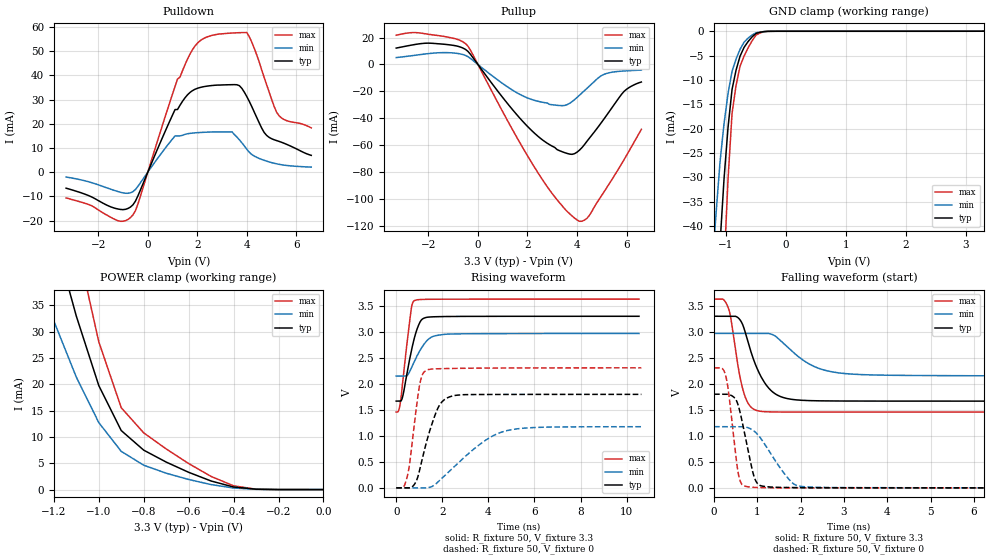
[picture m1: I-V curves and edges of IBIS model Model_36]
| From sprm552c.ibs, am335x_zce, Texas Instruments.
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| Model based on original model for BC1833DV50BPBFBP18LL_SSDHV
|   Sub model BC50B_V_PUPDOFF_10P_3P3
[model]   Model_36
|[Description]  [3.3V-I/O-PI-NORMAL, IND, 10%]
|   NORMAL,Weak pull up/down disabled,Industrial temperature range
|   (-40C to 125C, 25C nominal),10% power supply tolerance
|[Input Load]   PI
|[Output Drive] NORMAL
|Voltage   3.3V
|Mode   I/O
Model_type   I/O
Polarity   Non-Inverting
Enable   Active-Low
Vinl =  0.8V
Vinh =  2V
Cref =  15pF
Rref =  100.0000M
Vref =  0V
Vmeas =  1.65
C_comp   1.841028p   1.702526p   1.921952p
[Model Spec]
Vinl   0.8V   0.8V   0.8V
Vinh   2V   2V   2V
[Temperature Range]   25   125   -40
[Voltage Range]   3.3   2.97   3.63
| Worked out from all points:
|   slope of the pulldown table from 0 to 0.495 V, typ, clamps not added: 41.2 ohm
|   slope of the pullup table from 0 to 0.495 V, typ, clamps not added: 40 ohm
|   GND clamp passes 1 mA (typ) near -0.55 V on its own axis
|   POWER clamp passes 1 mA (typ) near -0.44 V on its own axis
|   rising waveform, R_fixture 50, V_fixture 3.3: 20-80 % time 461ps typ, 616ps min, 332ps max; typ from 1.67 V to 3.3 V
|   rising waveform, R_fixture 50, V_fixture 0: 20-80 % time 692ps typ, 1.86ns min, 386ps max; typ from 0 V to 1.8 V
|   falling waveform, R_fixture 50, V_fixture 3.3: 20-80 % time 464ps typ, 800ps min, 265ps max; typ from 3.3 V to 1.67 V
|   falling waveform, R_fixture 50, V_fixture 0: 20-80 % time 273ps typ, 571ps min, 191ps max; typ from 1.8 V to 0 V
[POWER_clamp]
-3.3V     437.1mA    413.2mA    590.8mA
-1.267V   59.46mA    39.86mA    84.25mA
-1.233V   53.93mA    35.93mA    76.6mA
-1.133V   38.09mA    24.91mA    54.45mA
-1.067V   28.54mA    18.48mA    40.82mA
-1.033V   24.14mA    15.6mA     34.44mA
-1V       19.75mA    12.72mA    28.06mA
-900mV    11.21mA    7.259mA    15.54mA
-800mV    7.487mA    4.633mA    10.77mA
-600mV    3.284mA    1.922mA    4.945mA
-400mV    494.5uA    303.8uA    719.2uA
0V        4.588uA    2.009uA    9.299uA
[Pulldown]
-3.3V     -6.622mA   -2.021mA   -10.65mA
-1.2V     -15.24mA   -8.032mA   -20.09mA
-600mV    -13.5mA    -8.05mA    -17.67mA
1.1V      25.87mA    14.97mA    35.44mA
1.2V      25.9mA     14.97mA    38.5mA
1.9V      34.23mA    16.24mA    52.08mA
2.5V      35.71mA    16.58mA    56.26mA
3.4V      36.16mA    16.66mA    57.51mA
4V        31.2mA     9.437mA    57.7mA
4.7V      16.38mA    4.891mA    39.13mA
5.2V      13.06mA    3.458mA    24.8mA
6.6V      6.944mA    2.091mA    18.31mA
[Pullup]
-3.3V     12.22mA    5.124mA    21.79mA
-2V       15.88mA    8.101mA    22.51mA
-500mV    11.19mA    6.71mA     15.51mA
1.4V      -33.67mA   -19.12mA   -48.63mA
2.4V      -53.04mA   -27.26mA   -79.87mA
3.5V      -65.59mA   -30.5mA    -107.4mA
3.8V      -66.88mA   -27.67mA   -112.7mA
4.1V      -63.77mA   -22.88mA   -116.7mA
4.4V      -57.22mA   -17.81mA   -114.5mA
5.1V      -40.3mA    -7.267mA   -94.57mA
5.9V      -20.05mA   -4.823mA   -70.85mA
6.6V      -13.04mA   -4.182mA   -48.28mA
[GND_clamp]
-3.3V     -759.3mA   -592.9mA   -1.187A
-1.233V   -79.57mA   -48.75mA   -128.9mA
-1.167V   -61.05mA   -37.35mA   -98.95mA
-1.1V     -43.5mA    -26.72mA   -70.29mA
-1.033V   -30.2mA    -18.9mA    -48.08mA
-966.7mV  -19.68mA   -12.74mA   -30.27mA
-900mV    -11.93mA   -8.215mA   -16.85mA
-833.3mV  -7.988mA   -5.689mA   -11.11mA
-766.7mV  -5.117mA   -3.7mA     -7.197mA
-700mV    -3.311mA   -2.248mA   -5.106mA
-500mV    -444.3uA   -319.3uA   -780.9uA
3.3V      4.588uA    93.88uA    5.606uA
[Ramp]
dV/dt_f   0.982646/0.4641994n 0.49553345/0.8052326n  1.3068592/0.26526249n
dV/dt_r  1.0820134/0.69291004n 0.70882467/1.870156n   1.3892168/0.38743151n
R_load = 50
[Rising Waveform]
R_fixture = 50
V_fixture = 3.3
V_fixture_min = 2.97
V_fixture_max = 3.63
0s        1.669V     2.15V      1.458V
138ps     1.669V     2.15V      1.536V
268ps     1.734V     2.15V      1.969V
468.4ps   2.203V     2.156V     2.78V
647.5ps   2.613V     2.295V     3.425V
798.1ps   2.899V     2.441V     3.602V
1.143ns   3.249V     2.722V     3.624V
1.511ns   3.288V     2.895V     3.627V
2.056ns   3.295V     2.95V      3.629V
10.54ns   3.3V       2.969V     3.63V
[Rising Waveform]
R_fixture = 50
V_fixture = 0
V_fixture_min = 0
V_fixture_max = 0
0s        0V         0V         0V
300ps     0V         0V         3.303mV
470.7ps   0V         0V         202.8mV
791.3ps   67.96mV    0V         1.242V
1.011ns   332.9mV    0V         1.966V
1.318ns   888.1mV    0V         2.265V
1.864ns   1.579V     135.3mV    2.291V
2.476ns   1.771V     392.1mV    2.297V
4.861ns   1.797V     1.107V     2.306V
10.64ns   1.798V     1.176V     2.308V
[Falling Waveform]
R_fixture = 50
V_fixture = 3.3
V_fixture_min = 2.97
V_fixture_max = 3.63
0s        3.3V       2.971V     3.629V
332.6ps   3.3V       2.971V     3.45V
590.6ps   3.24V      2.971V     2.165V
765.6ps   2.858V     2.971V     1.656V
1.008ns   2.267V     2.971V     1.482V
1.259ns   1.92V      2.968V     1.461V
1.561ns   1.747V     2.81V      1.458V
2.245ns   1.677V     2.36V      1.458V
2.979ns   1.67V      2.201V     1.457V
10.54ns   1.668V     2.151V     1.457V
[Falling Waveform]
R_fixture = 50
V_fixture = 0
V_fixture_min = 0
V_fixture_max = 0
0s        1.801V     1.176V     2.308V
268.9ps   1.801V     1.176V     2.155V
340.7ps   1.795V     1.176V     1.803V
552.6ps   1.6V       1.176V     304.2mV
720.2ps   984mV      1.172V     29.99mV
902.9ps   273.5mV    1.105V     10.14mV
1.018ns   68.54mV    1.015V     6.662mV
1.715ns   7.158mV    176.2mV    0V
2.011ns   4.122mV    28.03mV    0V
10.64ns   0V         0V         0V
